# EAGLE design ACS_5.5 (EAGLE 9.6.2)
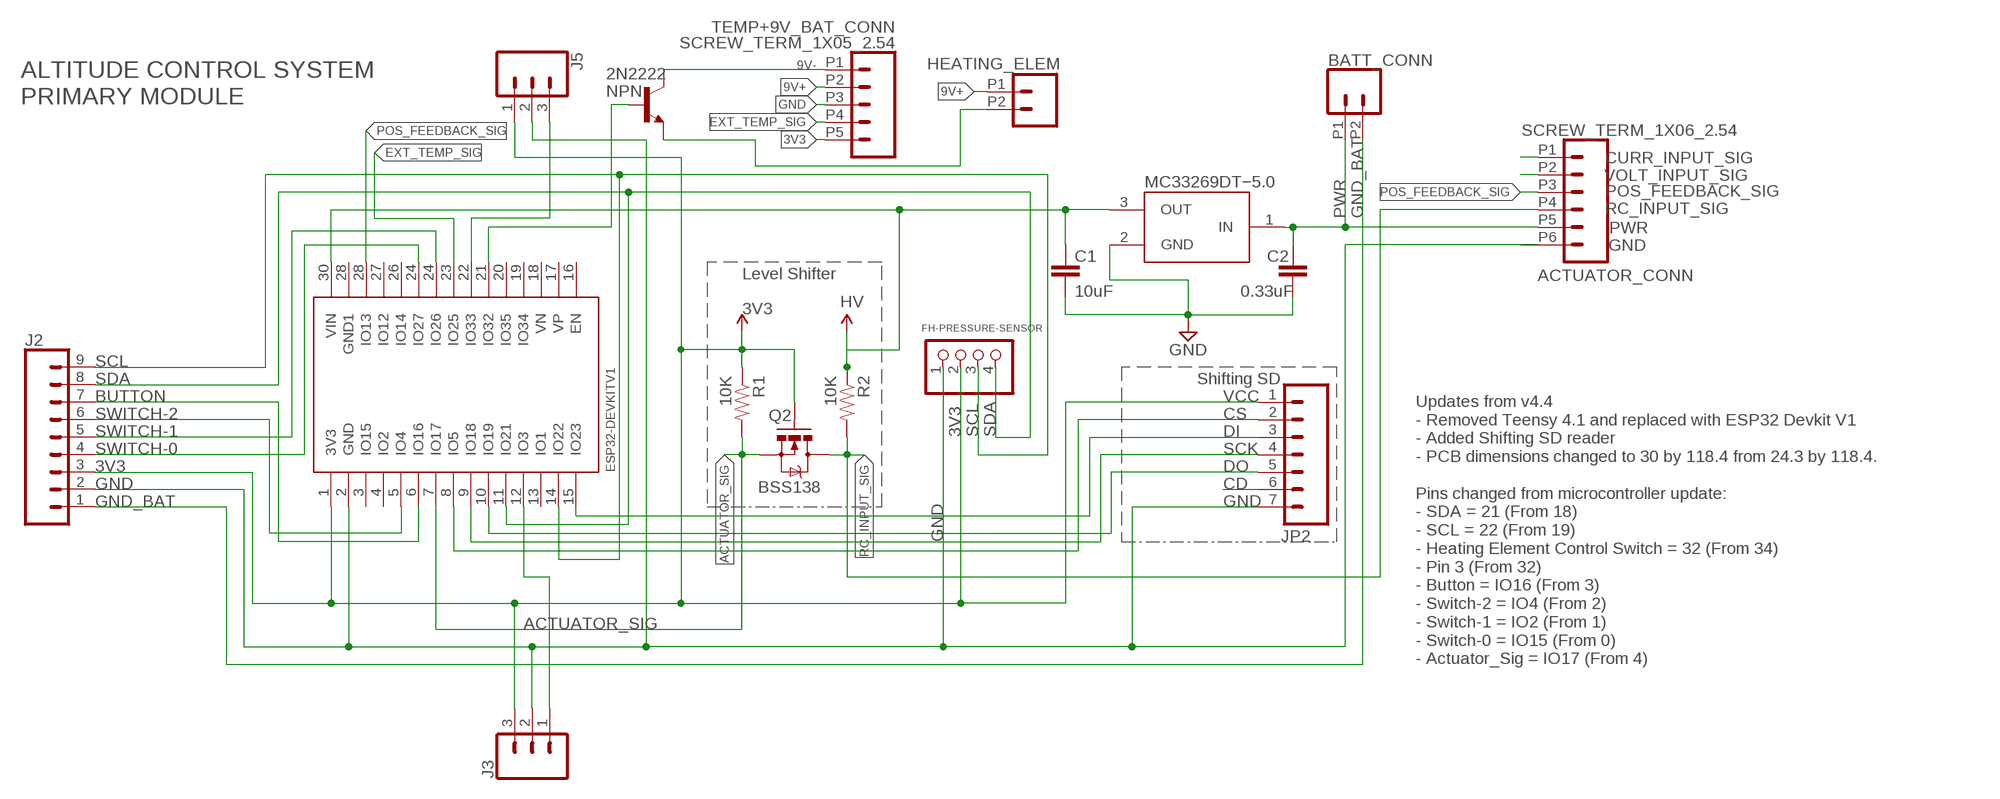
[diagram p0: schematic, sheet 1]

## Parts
2N2222  NPN  NPN_SOT23  [SOT95P237X112-3N]
ACTUATOR_CONN  SCREW_TERM_1X06_2.54  [1X06_2.54_SCREWTERM]
BATT_CONN  CONN_022.54MM_SCREWTERM  [1X02_2.54_SCREWTERM]
C1  10uF  C_CHIP-0603(1608-METRIC)  [CAPC1608X85]
C2  0.33uF  C_CHIP-0603(1608-METRIC)  [CAPC1608X85]
FH-PRESSURE-SENSOR  PINHD-1X4  [1X04]
HEATING_ELEM  CONN_022.54MM_SCREWTERM  [1X02_2.54_SCREWTERM]
J2  CONN_09  [1X09]
J3  CONN_03  [1X03]
J5  CONN_03  [1X03]
JP2  M07  [1X07]
Q2  BSS138  MOSFET-NCHANNELSMD  [SOT23-3]
R1  10K  RESISTOR0603-RES  [0603-RES]
R2  10K  RESISTOR0603-RES  [0603-RES]
TEMP+9V_BAT_CONN  SCREW_TERM_1X05_2.54  [1X05_2.54_SCREWTERM]
U1  MC78M05BDTRKG  [MC78M05BDTRKG]
U$3  ESP32DEVKITV1  [ESP32-DEVKITV1]

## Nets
3V3: FH-PRESSURE-SENSOR.2 J2.3 J3.3 J5.1 JP2.1 Q2.1(G) R1.1 TEMP+9V_BAT_CONN.P5 U$3.1(3V3) ; supply symbol labelled LV
9V+: HEATING_ELEM.P1 TEMP+9V_BAT_CONN.P2
9V-: 2N2222.3(C) TEMP+9V_BAT_CONN.P1
ACTUATOR_SIG: Q2.2(S) R1.2 U$3.7(IO17)
BUTTON: J2.7 U$3.6(IO16)
CURR_INPUT_SIG: ACTUATOR_CONN.P1
EXT_TEMP_SIG: TEMP+9V_BAT_CONN.P4 U$3.23(IO25)
GND: ACTUATOR_CONN.P6 C1.2 C2.2 FH-PRESSURE-SENSOR.1 J2.2 J3.2 J5.2 JP2.7 TEMP+9V_BAT_CONN.P3 U1.2(GND) U$3.2(GND)
GND_BAT: BATT_CONN.P2 J2.1
HV: C1.1 R2.1 U1.3(OUT) U$3.30(VIN)
N$1: J5.3 U$3.22(IO33)
N$5: 2N2222.2(B) U$3.21(IO32)
N$8: JP2.6
N$10: J3.1 U$3.12(IO3)
N$11: JP2.3 U$3.15(IO23)
N$12: JP2.2 U$3.8(IO5)
N$13: JP2.4 U$3.9(IO18)
N$14: JP2.5 U$3.10(IO19)
N$16: 2N2222.1(E) HEATING_ELEM.P2
POS_FEEDBACK_SIG: ACTUATOR_CONN.P3 U$3.28(IO13)
PWR: ACTUATOR_CONN.P5 BATT_CONN.P1 C2.1 U1.1(IN)
RC_INPUT_SIG: ACTUATOR_CONN.P4 Q2.3(D) R2.2
SCL: FH-PRESSURE-SENSOR.3 J2.9 U$3.14(IO22)
SDA: FH-PRESSURE-SENSOR.4 J2.8 U$3.11(IO21)
SWITCH-0: J2.4 U$3.24(IO27)
SWITCH-1: J2.5 U$3.24(IO26)
SWITCH-2: J2.6 U$3.5(IO4)
VOLT_INPUT_SIG: ACTUATOR_CONN.P2
Unconnected: U$3.3(IO15) U$3.4(IO2) U$3.13(IO1) U$3.16(EN) U$3.17(VP) U$3.18(VN) U$3.19(IO34) U$3.20(IO35) U$3.26(IO14) U$3.27(IO12) U$3.28(GND1)

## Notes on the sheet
- Heating Element 
  Control Switch
- ALTITUDE CONTROL SYSTEM
  PRIMARY MODULE
- Actuator Voltage: 7.5 MAX
- MC33269DT−5.0
- Level Shifter
- Shifting SD
- VCC
- CS
- DI
- SCK
- DO
- CD
- Updates from v4.4
  - Removed Teensy 4.1 and replaced with ESP32 Devkit V1
  - Added Shifting SD reader
  - PCB dimensions changed to 30 by 118.4 from 24.3 by 118.4.
  
  Pins changed from microcontroller update:
  - SDA = 21 (From 18)
  - SCL = 22 (From 19)
  - Heating Element Control Switch = 32 (From 34)
  - Pin 3 (From 32)
  - Button = IO16 (From 3)
  - Switch-2 = IO4 (From 2)
  - Switch-1 = IO2 (From 1)
  - Switch-0 = IO15 (From 0)
  - Actuator_Sig = IO17 (From 4)

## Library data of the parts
2N2222 = Transistor:NPN: NPN - Generic; CATEGORY: Transistor; SUB-CATEGORY: BJT; TYPE: NPN
ACTUATOR_CONN = Connectors-Terminal_Block:SCREW_TERM_1X06_2.54
BATT_CONN HEATING_ELEM = SparkFun-Connectors:CONN_02: Multi connection point. Often used as Generic Header-pin footprint for 0.1 inch spaced/style header connections
C1 C2 = Capacitor:C: Capacitor - Generic; CATEGORY: Capacitor
FH-PRESSURE-SENSOR = pinhead:PINHD-1X4: PIN HEADER
J2 = SparkFun-Connectors:CONN_09: Multi connection point. Often used as Generic Header-pin footprint for 0.1 inch spaced/style header connections On any of the 0.1 inch spaced packages, you can populate with these: Break Away Headers - Straight (PRT-00116) Break Away Male Headers - Right Angle (PRT-00553) Female Headers (PRT-00115)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
J3 J5 = SparkFun-Connectors:CONN_03: Multi connection point. Often used as Generic Header-pin footprint for 0.1 inch spaced/style header connections On any of the 0.1 inch spaced packages, you can populate with these: Break Away Headers - Straight (PRT-00116) Break Away Male Headers - Right Angle (PRT-00553) Female Headers (PRT-00115)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
JP2 = SparkFun-Connectors:M07: Header 7 Standard 7-pin 0.1" header. Use with straight break away headers (SKU : PRT-00116), right angle break away headers (PRT-00553), swiss pins (PRT-00743), machine pins (PRT-00117), and female headers (PRT-00115). NOTES ON THE VARIANTS LOCK and LOCK_LONGPADS... This footprint was designed to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
Q2 = SparkFun:MOSFET-NCHANNEL
R1 R2 = SparkFun:RESISTOR: Resistor
TEMP+9V_BAT_CONN = Connectors-Terminal_Block:SCREW_TERM_1X05_2.54
U1 = LDO:MC78M05BDTRKG: IC REG LINEAR 5V 500MA DPAK Manufacturer's datasheet; CREATED_BY: PCBLayout.com; DIGIKEY_PN: MC78M05BDTRKGOSCT-ND; MANUFACTURER: ON Semiconductor; MPN: IC REG LINEAR 5V 500MA DPAK; PACKAGE: DPak
U$3 = ESP32-DEVKITV1:ESP32DEVKITV1

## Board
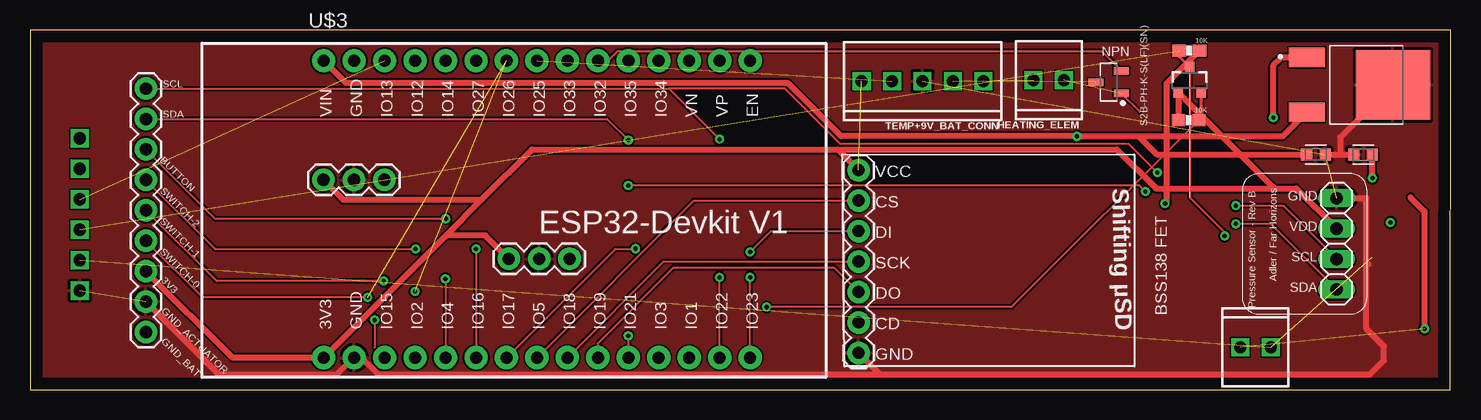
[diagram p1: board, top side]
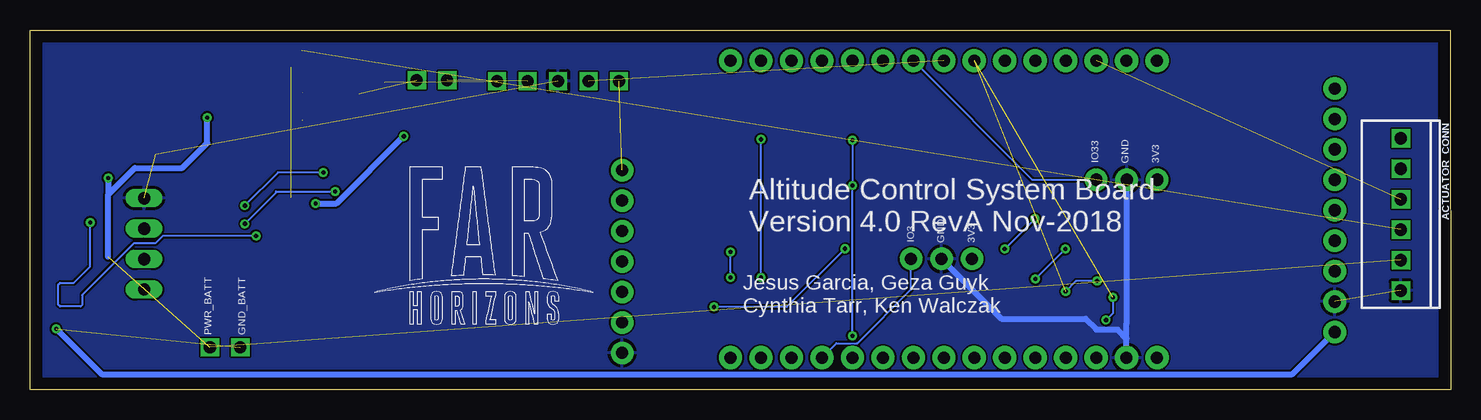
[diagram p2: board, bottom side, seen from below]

Size 118.43 x 30 mm. Coordinates in mm from the lower left corner, seen from the top.
Outline: 0,0 118.4,0 118.43,30 0.03,30 0,0
Copper layers (1*16): Top 0.035mm / dielectric 1.5mm / Bottom 0.035mm
Design rules "default": minimum track width 6mil, minimum drill 0.35mm, track to track 6mil, track to pad 6mil, pad to pad 6mil, via to via 6mil, smd to smd 6mil, copper to edge 40mil, drill to drill 6mil, minimum pad ring 10mil, minimum via ring 8mil, stop-mask expansion 4mil, vias tented up to drill 0mil, thermal gap 10mil

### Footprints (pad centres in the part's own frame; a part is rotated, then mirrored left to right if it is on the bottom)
SOT95P237X112-3N = smd 1.224 x 0.625: 1 -1.064,0.95; 2 -1.064,-0.95; 3 1.064,0
1X06_2.54_SCREWTERM = drill 1.016 square: P1 0,0; P2 2.54,0; P3 5.08,0; P4 7.62,0; P5 10.16,0; P6 12.7,0
1X02_2.54_SCREWTERM = drill 1.016 square: P1 2.54,0; P2 0,0
CAPC1608X85 = smd 0.921 x 0.97: 1 -0.775,0; 2 0.775,0
1X04 = drill 1.016 long: 1 -3.81,0; 2 -1.27,0; 3 1.27,0; 4 3.81,0
1X09 = drill 1.016 pad 1.88: 1 0,0; 2 2.54,0; 3 5.08,0; 4 7.62,0; 5 10.16,0; 6 12.7,0; 7 15.24,0; 8 17.78,0; 9 20.32,0
1X03 = drill 1.016 pad 1.88: 1 0,0; 2 2.54,0; 3 5.08,0
1X07 = drill 1.016 pad 1.88: 1 0,0; 2 2.54,0; 3 5.08,0; 4 7.62,0; 5 10.16,0; 6 12.7,0; 7 15.24,0
SOT23-3 = smd 0.8 x 0.9: 1 -0.95,-1; 2 0.95,-1; 3 0,1.1
0603-RES = smd 1.1 x 1: 1 -0.85,0; 2 0.85,0
1X05_2.54_SCREWTERM = drill 1.016 square: P1 0,0; P2 2.54,0; P3 5.08,0; P4 7.62,0; P5 10.16,0
MC78M05BDTRKG = smd 1.6 x 3: 1 -2.285,-4.08; 3 2.285,-4.08 | smd 5.8 x 6.2: 2 0,3.1
ESP32-DEVKITV1 = drill 1 pad 1.93: 1 -22.87,-13.54; 2 -20.33,-13.54; 3 -17.79,-13.54; 4 -15.25,-13.54; 5 -12.71,-13.54; 6 -10.17,-13.54; 7 -7.63,-13.54; 8 -5.09,-13.54; 9 -2.55,-13.54; 10 -0.01,-13.54; 11 2.53,-13.54; 12 5.07,-13.54; 13 7.61,-13.54; 14 10.15,-13.54; 15 12.69,-13.54; 16 12.69,11.23; 17 10.15,11.23; 18 7.61,11.23; 19 5.07,11.23; 20 2.53,11.23; 21 -0.01,11.23; 22 -2.55,11.23; 23 -5.09,11.23; 24 -7.63,11.23; 25 -10.17,11.23; 26 -12.71,11.23; 27 -15.25,11.23; 28 -17.79,11.23; 29 -20.33,11.23; 30 -22.87,11.23

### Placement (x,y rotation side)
2N2222  89.92,25.64 180 top
ACTUATOR_CONN  4.15,20.95 270 bottom
BATT_CONN  100.9,3.53 0 top
C1  107.19,19.61 0 top
C2  111.13,19.6 180 top
FH-PRESSURE-SENSOR  108.92,12.15 270 top
HEATING_ELEM  86.19,25.81 180 top
J2  9.66,4.79 90 top
J3  44.98,10.9 180 top
J5  24.46,17.5 0 top
JP2  69.07,18.3 270 top
Q2  96.67,25.79 0 top
R1  96.58,22.48 0 top
R2  96.64,28.28 180 top
TEMP+9V_BAT_CONN  79.48,25.73 180 top
U1  110.51,25.42 270 top
U$3  47.34,16.2 0 top

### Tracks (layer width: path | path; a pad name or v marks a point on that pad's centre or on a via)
3V3  (3 unrouted)
  Top 0.152: R1.1
  Top 0.254: 95.7,24.81 Q2.1
  Top 0.508: J2.3 16.88,2.65 U$3.1 34.67,12.86 | 34.67,12.86 37.66,15.85 | 37.66,15.85 41.84,20.03 67.34,20.03 | JP2.1 67.34,20.03 | 67.34,20.03 90.6,20.03 93.84,16.79 93.84,16.78 103.72,16.78 | 103.72,16.78 105.56,16.78 FH-PRESSURE-SENSOR.2 | R1.1 | 95.71,24.78 95.71,22.49 | J5.1 26.11,15.85 37.66,15.85 | J3.3 37.94,12.86 34.67,12.86 | 103.72,16.78 95.7,24.81
9V+  (1 unrouted)
9V-  (1 unrouted)
ACTUATOR_SIG  (via drill 0.35)
  Top 0.152: 97.5,22.55 R1.2 81.83,6.88 v61.41,6.88 | U$3.7 48.8,11.75 v50.48,11.75
  Top 0.254: Q2.2 97.62,22.67 97.5,22.55
  Bottom 0.152: v50.48,11.75 55.35,6.88 v61.41,6.88
BUTTON  (via drill 0.35)
  Top 0.152: v37.17,11.74 U$3.6 | v34.66,14.25 15.44,14.25 J2.7
  Bottom 0.152: v34.66,14.25 v37.17,11.74
EXT_TEMP_SIG  (1 unrouted)
GND  (3 unrouted)
  Top 0.508: C1.2 109.22,19.61 | 109.22,19.61 110.34,19.61 C2.2 | 109.22,19.61 109.22,21.03 U1.2 | J2.2 15.73,1.27 25.62,1.27 U$3.2 27.61,2.67 29.01,1.27 70.86,1.27 | 70.86,1.27 111.7,1.27 112.86,2.43 112.86,3.6 111.4,5.06 111.4,10.61 | JP2.7 70.86,1.27 | 111.56,10.45 111.4,10.61 | 111.4,10.61 111.4,15.95 111.39,15.96 FH-PRESSURE-SENSOR.1
  Bottom 0.508: U$3.2 27.02,4.25 | 27.02,4.25 27.02,5.51 27,5.53 J5.2 | J3.2 37.43,5.9 30.44,5.9 29.55,5.01 27.77,5.01 27.02,4.25
  pour Top: -4.15,31.64 -4.15,-1.81 119.4,-1.81 119.4,31.64
  pour Bottom: -5.76,31.6 -5.76,-1.75 119.61,-1.75 119.61,31.6
GND_BAT  (via drill 0.35)  (1 unrouted)
  Top 0.508: 115.07,16.04 116.25,14.86 v116.25,5.07 v116.25,5.06
  Bottom 0.508: v116.25,5.06 112.46,1.27 13.18,1.27 J2.1
HV  (via drill 0.35)
  Top 0.508: 24.48,27.43 26.31,25.6 63.13,25.6 67.61,21.13 v87.27,21.13 92.41,21.13 | 24.48,27.43 | U$3.30 24.48,27.43 | v94.62,15.52 94.75,15.65 94.75,25.53 R2.1 | 92.41,21.13 93.93,19.61 C1.1 | 92.41,21.13 104.42,21.13 U1.3
  Bottom 0.508: v94.62,15.52 92.88,15.52 v87.27,21.13
N$1
  Bottom 0.152: J5.3 34.86,17.5 U$3.22
N$5
  Top 0.152: U$3.21 48.19,27.43 48.97,28.22 89.36,28.22 2N2222.2
N$10
  Bottom 0.152: U$3.12 51.22,3.86 49.46,3.86 44.98,8.35 J3.1
N$11  (via drill 0.35)
  Top 0.152: U$3.15 v60.03,9.35 | v60.03,11.48 61.77,13.22 JP2.3
  Bottom 0.152: v60.03,9.35 v60.03,11.48
N$12
  Top 0.152: U$3.8 55.35,15.76 JP2.2
N$13
  Top 0.152: U$3.9 52.81,10.68 JP2.4
N$14
  Top 0.152: U$3.10 47.34,3.85 53.61,10.13 67.08,10.13 JP2.5
N$16  (1 unrouted)
  Top 0.152: 2N2222.1 92.5,23.17
POS_FEEDBACK_SIG  (1 unrouted)
PWR  (via drill 0.35)  (2 unrouted)
  Top 0.508: v111.91,17.65 C2.1 | U1.1 104.3,27.7 103.65,27.06 v103.65,22.68
  Bottom 0.508: 111.91,11.07 111.91,16.27 | v111.91,17.65 111.91,16.27 | 111.91,16.27 109.69,18.49 105.74,18.49 103.65,20.58 v103.65,22.68
RC_INPUT_SIG  (via drill 0.35)  (2 unrouted)
  Top 0.152: Q2.3 96.67,16.01 99.59,13.1 v99.59,12.82
  Top 0.254: R2.2 95.79,27.77 Q2.3
  Bottom 0.152: v99.59,12.82 107.36,12.82 107.98,12.2 109.76,12.2 114.08,7.89 114.08,7.05 114.21,6.92 115.93,6.92 116.06,7.05 116.06,8.76 115.93,8.9 114.77,8.9 113.41,10.26 v113.41,13.94
SCL  (via drill 0.35)
  Top 0.152: U$3.14 v57.49,9.35 v57.49,9.36 | J2.9 53.25,25.11 | 53.25,25.11 v57.49,20.88 | v93.98,18.11 91.56,20.52 67.53,20.52 62.94,25.11 53.25,25.11 | v100.52,15.34 104.46,15.34 FH-PRESSURE-SENSOR.3
  Bottom 0.152: v93.98,18.11 97.75,18.11 v100.52,15.34 | v57.49,9.36 v57.49,20.88
SDA  (via drill 0.35)
  Top 0.152: J2.8 48.12,22.57 | v92.98,16.53 92.48,17.03 v49.88,17.03 | FH-PRESSURE-SENSOR.4 103.43,13.83 v100.52,13.83 | v49.88,20.82 48.12,22.57 | 48.12,22.57 | U$3.11 v49.88,4.49
  Bottom 0.152: v100.52,13.83 97.91,16.44 97.91,16.53 v92.99,16.53 v92.98,16.53 | v49.88,20.82 v49.88,17.03 v49.88,4.49
SWITCH-0  (via drill 0.35)  (1 unrouted)
  Top 0.152: v28.16,7.7 14.38,7.7 J2.4 | v28.73,5.8 28.71,5.79 28.71,3.5
  Bottom 0.152: v28.73,5.8 28.18,6.34 28.18,7.68 v28.16,7.7
SWITCH-1  (via drill 0.35)  (1 unrouted)
  Top 0.152: v29.47,9.06 15.55,9.06 J2.5
  Bottom 0.152: v29.47,9.06 31.23,9.06 v32.09,8.19
SWITCH-2  (via drill 0.35)
  Top 0.152: v34.62,9.23 34.62,2.67 U$3.5 | J2.6 15.43,11.72 v32.13,11.72
  Bottom 0.152: v34.62,9.23 v32.13,11.72

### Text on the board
tPlace: Shifting µSD
bPlace: Altitude Control System Board / Version 4.0 RevA Nov-2018 | Jesus Garcia, Geza Guyk / Cynthia Tarr, Ken Walczak
tNames: 10K | NPN | SCL | SDA | 10K | S2B-PH-K-S(LF)(SN) | BUTTON | VCC | SWITCH-2 | Pressure Sensor - Rev B | Adler / Far Horizons | GND | CS | SWITCH-1 | VDD | DI | SWITCH-0 | SCL | SCK | 3V3 | SDA | DO | GND_ACTUATOR | BSS138 FET | CD | GND_BAT | GND
bNames: GND | IO33 | 3V3 | 3V3 | GND | IO3 | GND_BATT | PWR_BATT
tValues: 10uF | 0.33uF

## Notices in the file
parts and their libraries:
SparkFun-Connectors: Licensing: Creative Commons ShareAlike 4.0 International - https://creativecommons.org/licenses/by-sa/4.0
SparkFun-Connectors: Licensing: CC v3.0 Share-Alike You are welcome to use this library for commercial purposes.
